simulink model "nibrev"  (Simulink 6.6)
settings: Solver=ode45  StartTime=0.0  StopTime=25.0  RelTol=1e-3
undefined symbols (not defined in the file or in its folder): Bit, Location, Lower, netlist, Width
libraries: xbsIndex_r4 x17, adlibrary2 x1

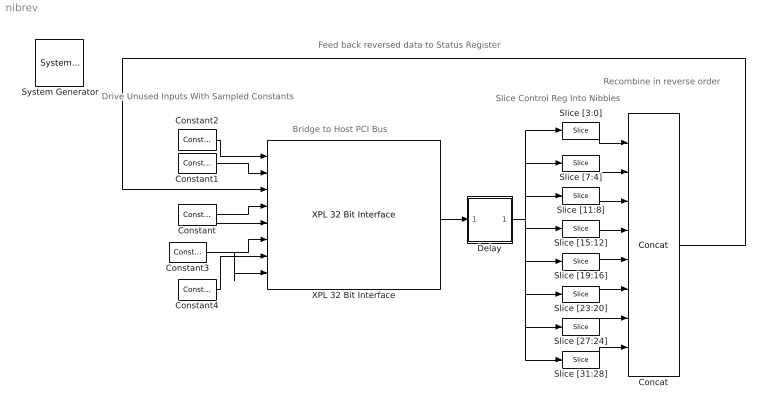
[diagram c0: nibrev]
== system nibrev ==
  note: Drive Unused Inputs With Sampled Constants
  note: Bridge to Host PCI Bus
  note: Slice Control Reg Into Nibbles
  note: Recombine in reverse order
  note: Feed back reversed data to Status Register
  " System Generator" : xbsIndex_r4/ System Generator  Tag=genX  SystemSampleTime=-1  xilinxfamily=virtex5  part=xc5vlx330t  speed=-1  package=ff1738  synthesis_tool=XST  directory=./netlist  testbench=off  simulink_period=1  sysclk_period=10  incr_netlist=off  trim_vbits=Everywhere in SubSystem  dbl_ovrd=According to Block Masks  core_generation=According to Block Masks  run_coregen=off  deprecated_control=off  eval_field=0  block_type=sysgen
  Concat : xbsIndex_r4/Concat  num_inputs=8  dbl_ovrd=off  block_type=concat
  Constant : xbsIndex_r4/Constant  arith_type=Boolean  const=0  n_bits=1  bin_pt=0  explicit_period=on  period=1  equ=P=C  opselect=C  inp2=PCIN>>17  opr=+  inp1=P  carry=CIN  dbl_ovrd=off  block_type=constant
  Constant1 : xbsIndex_r4/Constant  arith_type=Boolean  const=1  n_bits=1  bin_pt=0  explicit_period=on  period=1  equ=P=C  opselect=C  inp2=PCIN>>17  opr=+  inp1=P  carry=CIN  dbl_ovrd=off  block_type=constant
  Constant2 : xbsIndex_r4/Constant  arith_type=Unsigned  const=0  n_bits=32  bin_pt=0  explicit_period=on  period=1  equ=P=C  opselect=C  inp2=PCIN>>17  opr=+  inp1=P  carry=CIN  dbl_ovrd=off  block_type=constant
  Constant3 : xbsIndex_r4/Constant  arith_type=Unsigned  const=0  n_bits=32  bin_pt=0  explicit_period=on  period=1  equ=P=C  opselect=C  inp2=PCIN>>17  opr=+  inp1=P  carry=CIN  dbl_ovrd=off  block_type=constant
  Constant4 : xbsIndex_r4/Constant  arith_type=Unsigned  const=0  n_bits=66  bin_pt=0  explicit_period=on  period=1  equ=P=C  opselect=C  inp2=PCIN>>17  opr=+  inp1=P  carry=CIN  dbl_ovrd=off  block_type=constant
  Delay : Subsystem
  Slice [11:8] : xbsIndex_r4/Slice  nbits=4  boolean_output=off  mode=Lower Bit Location + Width  bit1=0  base1=MSB of Input  bit0=8  base0=LSB of Input  dbl_ovrd=off  block_type=slice
  Slice [15:12] : xbsIndex_r4/Slice  nbits=4  boolean_output=off  mode=Lower Bit Location + Width  bit1=0  base1=MSB of Input  bit0=12  base0=LSB of Input  dbl_ovrd=off  block_type=slice
  Slice [19:16] : xbsIndex_r4/Slice  nbits=4  boolean_output=off  mode=Lower Bit Location + Width  bit1=0  base1=MSB of Input  bit0=16  base0=LSB of Input  dbl_ovrd=off  block_type=slice
  Slice [23:20] : xbsIndex_r4/Slice  nbits=4  boolean_output=off  mode=Lower Bit Location + Width  bit1=0  base1=MSB of Input  bit0=20  base0=LSB of Input  dbl_ovrd=off  block_type=slice
  Slice [27:24] : xbsIndex_r4/Slice  nbits=4  boolean_output=off  mode=Lower Bit Location + Width  bit1=0  base1=MSB of Input  bit0=24  base0=LSB of Input  dbl_ovrd=off  block_type=slice
  Slice [31:28] : xbsIndex_r4/Slice  nbits=4  boolean_output=off  mode=Lower Bit Location + Width  bit1=0  base1=MSB of Input  bit0=28  base0=LSB of Input  dbl_ovrd=off  block_type=slice
  Slice [3:0] : xbsIndex_r4/Slice  nbits=4  boolean_output=off  mode=Lower Bit Location + Width  bit1=0  base1=MSB of Input  bit0=0  base0=LSB of Input  dbl_ovrd=off  block_type=slice
  Slice [7:4] : xbsIndex_r4/Slice  nbits=4  boolean_output=off  mode=Lower Bit Location + Width  bit1=0  base1=MSB of Input  bit0=4  base0=LSB of Input  dbl_ovrd=off  block_type=slice
  XPL 32 Bit Interface : adlibrary2/ADM-XPL/XPL 32 Bit Interface  SystemSampleTime=-1  program='load myprogram.txt'  clock_ratio=1.5  sstep_clk_sel_default=0
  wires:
  Constant/1 -> XPL 32 Bit Interface/4, XPL 32 Bit Interface/5
  Constant1/1 -> XPL 32 Bit Interface/2
  Constant2/1 -> XPL 32 Bit Interface/1
  Constant3/1 -> XPL 32 Bit Interface/8, XPL 32 Bit Interface/6
  Constant4/1 -> XPL 32 Bit Interface/7
  XPL 32 Bit Interface/6 -> Delay/1(in0)
  Delay/1(out0) -> Slice [31:28]/1, Slice [27:24]/1, Slice [23:20]/1, Slice [19:16]/1, Slice [15:12]/1, Slice [11:8]/1, Slice [3:0]/1, Slice [7:4]/1
  Slice [3:0]/1 -> Concat/1
  Slice [7:4]/1 -> Concat/2
  Slice [11:8]/1 -> Concat/3
  Slice [15:12]/1 -> Concat/4
  Slice [19:16]/1 -> Concat/5
  Slice [23:20]/1 -> Concat/6
  Slice [27:24]/1 -> Concat/7
  Slice [31:28]/1 -> Concat/8
  Concat/1 -> XPL 32 Bit Interface/3

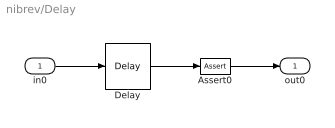
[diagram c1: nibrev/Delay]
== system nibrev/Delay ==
  in0 : Inport
  Assert0 : xbsIndex_r4/Assert  assert_type=off  type_source=Explicitly  arith_type="Signed  (2's comp)"  n_bits=16  bin_pt=14  assert_rate=on  rate_source=Explicitly  period=1  output_port=on  block_type=assert
  Delay : xbsIndex_r4/Delay  en=off  latency=1  dbl_ovrd=off  reg_retiming=off  block_type=delay
  out0 : Outport
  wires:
  in0/1 -> Delay/1
  Delay/1 -> Assert0/1
  Assert0/1 -> out0/1
